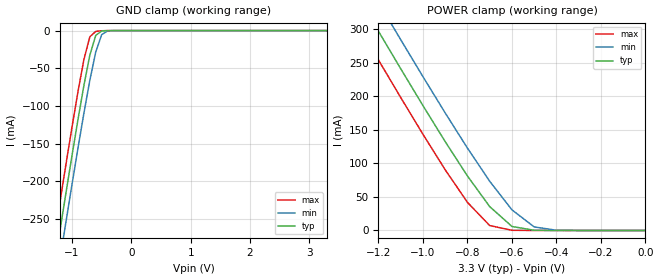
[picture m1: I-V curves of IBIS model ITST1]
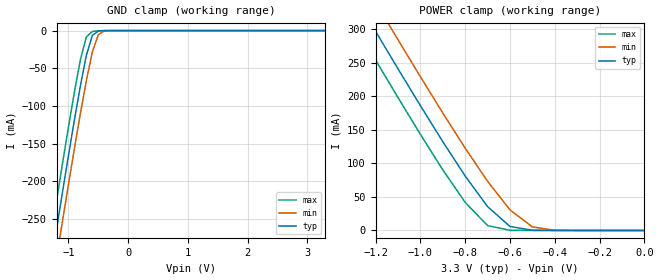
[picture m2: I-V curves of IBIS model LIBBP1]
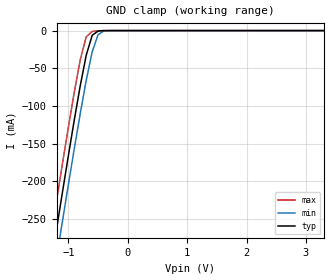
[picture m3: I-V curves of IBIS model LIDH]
[IBIS Ver]   2.1
[File name]   a22r1033.ibs
[File Rev]   1.0
[Date]   11/01/2002
[Source]   SEIKO EPSON Corp.
[Notes]
[Disclaimer]   Data is for modeling purposes only and is not guaranteed
   more disclaimer
[Copyright]   Copyright 2002 by ADTEK System Science Co.,Ltd.
[Component]   S1L53353F22P000
[Manufacturer] SEIKO EPSON Corp.
[Package]
|   QFP20-184
|   typ   min   max
R_pkg   53.7m   50.9m   56.3m
L_pkg   7.78nH   7.03nH   8.94nH
C_pkg   0.668pF  0.598pF  0.761pF
[Pin]  signal_name model_name
1 VSS GND
2 PB_CXBE3 HBPGT
3 PB_IDSEL HIBPG
4 PB_AD23 HBPGT
5 PB_AD22 HBPGT
6 PB_AD21 HBPGT
7 PB_AD20 HBPGT
8 HVDD POWER
9 VSS GND
10 PB_AD19 HBPGT
11 PB_AD18 HBPGT
12 PB_AD17 HBPGT
13 PB_AD16 HBPGT
14 HVDD POWER
15 VSS GND
16 PB_CXBE2 HBPGT
17 PB_XFRAME HBPGT
18 PB_XIRDY HBPGT
19 PB_XTRDY HBPGT
20 PB_XDVSEL HBPGT
21 PB_XSTOP HBPGT
22 LVDD POWER
23 VSS GND
24 PB_XLOCK HBPGT
25 PB_XPERR HBPGT
26 PB_XSERR HTBPCT
27 PB_PAR HBPGT
28 PB_CXBE1 HBPGT
29 HVDD POWER
30 VSS GND
31 PB_AD15 HBPGT
32 PB_AD14 HBPGT
33 PB_AD13 HBPGT
34 PB_AD12 HBPGT
35 HVDD POWER
36 VSS GND
37 PB_AD11 HBPGT
38 PB_AD10 HBPGT
39 PB_AD9 HBPGT
40 PB_AD8 HBPGT
41 PB_CXBE0 HBPGT
42 LVDD POWER
43 VSS GND
44 TEST LIDHD1
| 45 HVDCT HVDCT
46 HVDD POWER
47 VSS GND
48 PB_AD7 HBPGT
49 PB_AD6 HBPGT
50 PB_AD5 HBPGT
51 PB_AD4 HBPGT
52 HVDD POWER
53 VSS GND
54 PB_AD3 HBPGT
55 PB_AD2 HBPGT
56 PB_AD1 HBPGT
57 PB_AD0 HBPGT
58 HVDD POWER
59 VSS GND
60 PB_XENUM HBPGT
61 LVDD POWER
62 VSS GND
63 XLRESET LOB2T
64 LB_XBACK LOB2T
65 LB_XBREQ LIBBP2
66 LB_XDREQ LIBBP2
67 LB_XDACK LTBF2
68 LB_XDMATC LTBF2
69 LVDD POWER
70 VSS GND
71 LB_IORDY LBB2P2
72 LB_XIOW LBB2P2
73 LB_XIOR LBB2P2
74 LB_XMWR LBB2P2
75 LB_XMRD LBB2P2
76 LB_XMEMCS LTBF2
77 LB_XROMCS LTBF2
78 LVDD POWER
79 VSS GND
80 LB_IOCS0 LBB2P2
81 LB_IOCS1 LBB2P2
82 LB_IOCS2 LBB2P2
83 LB_IOCS3 LBB2P2
84 LB_IOCS4 LBB2P2
85 LB_IOCS5 LBB2P2
86 LB_IOCS6 LBB2P2
87 LB_IOCS7 LBB2P2
88 LB_XBHE LBB2P2
89 VSS GND
90 LCLKI LIBBP1
91 LCLKO LOB2T
92 LVDD POWER
93 VSS GND
94 LB_SPACE LIBBP2
95 LB_XDEVCS LIBBP2
96 NC NC
97 LVDD POWER
98 VSS GND
99 LB_AD0 LBB2P2
100 LB_AD1 LBB2P2
101 LB_AD2 LBB2P2
102 LB_AD3 LBB2P2
103 LB_AD4 LBB2P2
104 LB_AD5 LBB2P2
105 LB_AD6 LBB2P2
106 LB_AD7 LBB2P2
107 LVDD POWER
108 VSS GND
109 LB_AD8 LBB2P2
110 LB_AD9 LBB2P2
111 LB_AD10 LBB2P2
112 LB_AD11 LBB2P2
113 LB_AD12 LBB2P2
114 LB_AD13 LBB2P2
115 LB_AD14 LBB2P2
116 LB_AD15 LBB2P2
117 LVDD POWER
118 VSS GND
119 LB_AD16 LBB2P2
120 LB_AD17 LBB2P2
121 LB_AD18 LBB2P2
122 LB_AD19 LBB2P2
123 LB_AD20 LBB2P2
124 LB_AD21 LBB2P2
125 LB_AD22 LBB2P2
126 LB_AD23 LBB2P2
127 LVDD POWER
128 VSS GND
129 LB_AD24 LBB2P2
130 LB_AD25 LBB2P2
131 LB_AD26 LBB2P2
132 LB_AD27 LBB2P2
133 LB_AD28 LBB2P2
134 LB_AD29 LBB2P2
135 LB_AD30 LBB2P2
136 LB_AD31 LBB2P2
137 LB_A16 LBB2P2
138 LVDD POWER
139 VSS GND
140 IRQ3 LIBBP2
141 IRQ2 LIBBP2
142 IRQ1 LIBBP2
143 IRQ0 LIBBP2
144 XLINT LOD2T
145 XTOUT LTBF2
146 VSS GND
147 XEJECT LIDHD2
148 PB_XSTLED LOD3T
149 PIO3 LBB2P2
150 PIO2 LBB2P2
151 PIO1 LBB2P2
152 PIO0 LBB2P2
153 LVDD POWER
154 VSS GND
155 TSTEN ITST1
156 INP2 LIDHD2
157 INP1 LIDHD2
158 INP0 LIDHD2
159 EECS_SL LBG2D2
160 EESK LTBF2
161 EEDI LBG2
162 EEDO LIDH
163 XHELTHY LIDHD2
164 LVDD POWER
165 VSS GND
166 PB_XINTA HTBPCT
167 XRESET HIBPC
168 VSS GND
169 PCI_CLK HIBPC
170 PB_XGNT HIBPG
171 PB_XREQ HTBPCT
172 PB_XPME HTBPCT
173 VSS GND
174 PB_AD31 HBPGT
175 PB_AD30 HBPGT
176 PB_AD29 HBPGT
177 PB_AD28 HBPGT
178 HVDD POWER
179 VSS GND
180 PB_AD27 HBPGT
181 PB_AD26 HBPGT
182 PB_AD25 HBPGT
183 PB_AD24 HBPGT
184 HVDD POWER
| Models and submodels in the file (17): ITST1 (Input), LIBBP1 (Input), LIBBP2 (Input), LIDH (Input), LIDHD1 (Input), LIDHD2 (Input), HIBPC (Input), HIBPG (Input), LOB2T (Output), LOD2T (Output), LOD3T (Output), LTBF2 (Output), HTBPCT (Output), LBB2P2 (I/O), LBG2 (I/O), LBG2D2 (I/O), HBPGT (I/O)
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[Model]   ITST1
Model_type   Input
Polarity   Non-Inverting
Vinh=2.0V
Vinl=0.8V
|   typ   min   max
C_comp   5.0pF   4.0pF   6.0pF
|   typ   min   max
[Voltage range]   3.3   3.0   3.6
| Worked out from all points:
|   GND clamp passes 1 mA (typ) near -0.51 V on its own axis
|   POWER clamp passes 1 mA (typ) near -0.51 V on its own axis
[GND_clamp]
|   Voltage   I(typ)   I(min)   I(max)
-3.3V     -1.343A    -1.379A    -1.309A
-1.3V     -314.1mA   -352.4mA   -276.2mA
-1.2V     -264.1mA   -302.5mA   -226.1mA
-1.1V     -214.6mA   -253.1mA   -176.6mA
-1V       -165.9mA   -204.2mA   -128.1mA
-900mV    -118.4mA   -156.3mA   -81.33mA
-800mV    -73.08mA   -109.9mA   -38.6mA
-700mV    -32.75mA   -66.18mA   -8.318mA
-600mV    -6.318mA   -28.41mA   -1.129mA
-500mV    -586.9uA   -5.399mA   -239.5uA
-400mV    -56.77uA   -404.4uA   -18.72uA
3.3V      7.178nA    15.7uA     6.02nA
[POWER_clamp]
|   Voltage   I(typ)   I(min)   I(max)
-3.3V     1.514A     1.553A     1.476A
-1.3V     353.1mA    396.1mA    310.4mA
-1.2V     296.7mA    339.9mA    253.9mA
-1.1V     240.9mA    284.1mA    198mA
-1V       185.9mA    229mA      143.2mA
-900mV    132.3mA    175mA      90.33mA
-800mV    81.11mA    122.6mA    41.82mA
-700mV    35.52mA    73.27mA    7.314mA
-600mV    5.969mA    30.7mA     281.7uA
-500mV    284.1uA    5.285mA    30.01uA
-400mV    15.7uA     326.5uA    2.385uA
0V        7.178nA    15.84nA    7.223nA
[Model]   LIBBP1
Model_type   Input
Polarity   Non-Inverting
Vinh=2.0V
Vinl=0.8V
|   typ   min   max
C_comp   5.0pF   4.0pF   6.0pF
|   typ   min   max
[Voltage range]   3.3   3.0   3.6
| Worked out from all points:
|   GND clamp passes 1 mA (typ) near -0.51 V on its own axis
|   POWER clamp passes 1 mA (typ) near -0.51 V on its own axis
[GND_clamp]
|   Voltage   I(typ)   I(min)   I(max)
-3.3V     -1.343A    -1.379A    -1.309A
-1.3V     -314.1mA   -352.4mA   -276.2mA
-1.2V     -264.1mA   -302.5mA   -226.1mA
-1.1V     -214.6mA   -253.1mA   -176.6mA
-1V       -165.9mA   -204.2mA   -128.1mA
-900mV    -118.4mA   -156.3mA   -81.33mA
-800mV    -73.08mA   -109.9mA   -38.6mA
-700mV    -32.75mA   -66.18mA   -8.318mA
-600mV    -6.318mA   -28.41mA   -1.129mA
-500mV    -586.9uA   -5.399mA   -239.5uA
-400mV    -56.77uA   -404.4uA   -18.72uA
3.3V      7.252nA    15.71uA    5.938nA
[POWER_clamp]
|   Voltage   I(typ)   I(min)   I(max)
-3.3V     1.514A     1.553A     1.476A
-1.3V     353.1mA    396.1mA    310.4mA
-1.2V     296.7mA    339.9mA    253.9mA
-1.1V     240.9mA    284.1mA    198mA
-1V       185.9mA    229mA      143.2mA
-900mV    132.3mA    175mA      90.33mA
-800mV    81.11mA    122.6mA    41.82mA
-700mV    35.52mA    73.27mA    7.314mA
-600mV    5.969mA    30.7mA     281.7uA
-500mV    284.1uA    5.285mA    30.01uA
-400mV    15.7uA     326.5uA    2.386uA
0V        7.252nA    15.98nA    7.296nA
[Model]   LIDH
Model_type   Input
Polarity   Non-Inverting
Vinh=2.0V
Vinl=0.8V
|   typ   min   max
C_comp   5.0pF   4.0pF   6.0pF
|   typ   min   max
[Voltage range]   3.3   3.0   3.6
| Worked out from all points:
|   GND clamp passes 1 mA (typ) near -0.51 V on its own axis
[GND_clamp]
|   Voltage   I(typ)   I(min)   I(max)
-3.3V     -1.343A    -1.379A    -1.309A
-1.3V     -314.1mA   -352.4mA   -276.2mA
-1.2V     -264.1mA   -302.5mA   -226.1mA
-1.1V     -214.6mA   -253.1mA   -176.6mA
-1V       -165.9mA   -204.2mA   -128.1mA
-900mV    -118.4mA   -156.3mA   -81.33mA
-800mV    -73.08mA   -109.9mA   -38.6mA
-700mV    -32.75mA   -66.18mA   -8.318mA
-600mV    -6.318mA   -28.41mA   -1.129mA
-500mV    -586.9uA   -5.399mA   -239.5uA
-400mV    -56.77uA   -404.4uA   -18.72uA
3.3V      7.178nA    15.7uA     6.022nA
